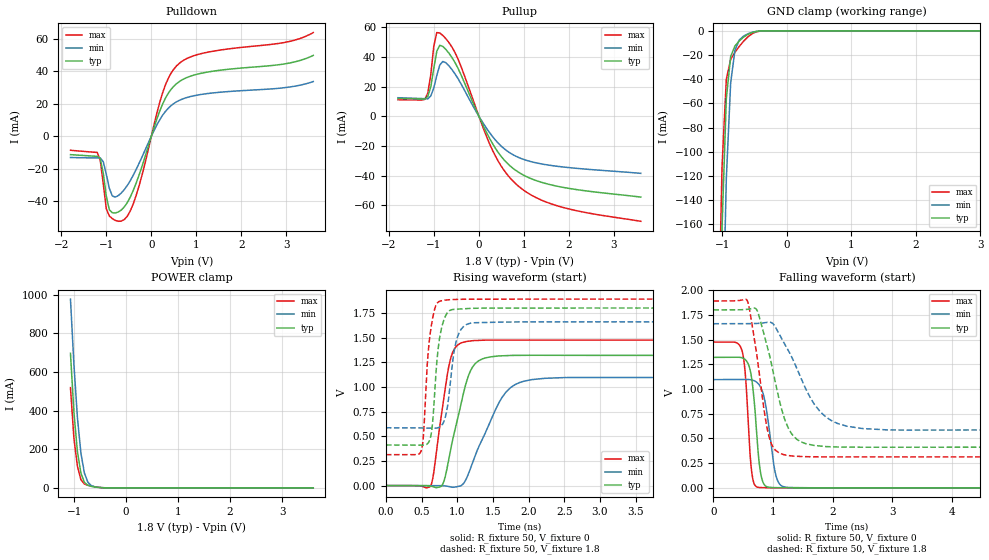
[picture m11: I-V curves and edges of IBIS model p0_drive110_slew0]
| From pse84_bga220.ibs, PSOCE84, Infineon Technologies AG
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[Model] p0_drive110_slew0
Model_type I/O
Polarity  Inverting
Enable   Active-High
Vinl  =  0.54
Vinh  =  1.26
Vmeas =  0.9
Cref  =  15pF
| Capacitance   typ   min   max
C_comp   1.253838e-12   1.215159e-12   1.300411e-12
| Variables   typ   min   max
[GND Clamp Reference]   0   0   0
[POWER Clamp Reference]   1.8   1.66   1.89
[Pulldown Reference]   0   0   0
[Pullup Reference]   1.8   1.66   1.89
[Temperature Range]   25   125   -40
[Voltage Range]   1.8   1.66   1.89
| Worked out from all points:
|   slope of the pulldown table from 0 to 0.27 V, typ, clamps not added: 12.9 ohm
|   slope of the pullup table from 0 to 0.27 V, typ, clamps not added: 16.3 ohm
|   GND clamp passes 1 mA (typ) near -0.51 V on its own axis
|   POWER clamp passes 1 mA (typ) near -0.47 V on its own axis
|   rising waveform, R_fixture 50, V_fixture 0: 20-80 % time 250ps typ, 406ps min, 174ps max; typ from 0 V to 1.32 V
|   rising waveform, R_fixture 50, V_fixture 1.8: 20-80 % time 98.2ps typ, 117ps min, 90.6ps max; typ from 0.411 V to 1.8 V
|   falling waveform, R_fixture 50, V_fixture 0: 20-80 % time 113ps typ, 152ps min, 89.3ps max; typ from 1.32 V to 0 V
|   falling waveform, R_fixture 50, V_fixture 1.8: 20-80 % time 335ps typ, 546ps min, 224ps max; typ from 1.8 V to 0.411 V
[GND Clamp]
| Voltage   I(typ)   I(min)   I(max)
-1.137V   -619.5mA   -754.2mA   -533mA
-1.07V    -361.2mA   -498.1mA   -281.3mA
-1.003V   -163.8mA   -277.7mA   -113mA
-936.6mV  -56.22mA   -122.3mA   -40.06mA
-869.7mV  -21.33mA   -43.3mA    -23.67mA
-802.8mV  -12.5mA    -15.96mA   -17.71mA
-735.9mV  -8.346mA   -7.675mA   -12.88mA
-669mV    -5.267mA   -4.349mA   -8.575mA
-535.2mV  -1.314mA   -1.207mA   -2.328mA
-401.4mV  -73.55uA   -132.2uA   -119.3uA
3.6V      0A         0A         0A
[POWER Clamp]
| Voltage   I(typ)   I(min)   I(max)
-1.07V    696.7mA    977.2mA    518.8mA
-1.003V   390.1mA    637.2mA    255.1mA
-936.6mV  187.1mA    363.9mA    112.4mA
-869.7mV  77.2mA     180.7mA    42.71mA
-802.8mV  28.89mA    77.43mA    19.98mA
-735.9mV  13.12mA    29.18mA    13.35mA
-669mV    7.754mA    11.55mA    8.954mA
-535.2mV  2.356mA    2.862mA    2.667mA
-334.5mV  34.33uA    127.4uA    15.58uA
3.6V      0A         0A         0A
[Pullup]
| Voltage   I(typ)   I(min)   I(max)
-1.8V     11.96mA    12.52mA    11.17mA
-1.204V   11.63mA    11.87mA    11.36mA
-1.07V    19.81mA    13.65mA    28.15mA
-1.003V   32.26mA    19.14mA    47.26mA
-936.6mV  43.85mA    27.48mA    56.38mA
-869.7mV  47.83mA    34.58mA    56.11mA
-735.9mV  45.06mA    36.08mA    52.29mA
-468.3mV  32.52mA    25.53mA    38.8mA
310.3mV   -18.74mA   -13.88mA   -23.33mA
806.9mV   -36.11mA   -26.63mA   -45.05mA
1.738V    -47.03mA   -33.62mA   -60.19mA
3.6V      -54.37mA   -38.39mA   -70.66mA
[Pulldown]
| Voltage   I(typ)   I(min)   I(max)
-1.8V     -11.4mA    -13.16mA   -8.708mA
-1.204V   -12.44mA   -13.38mA   -10.06mA
-1.137V   -13.75mA   -13.38mA   -14.91mA
-1.003V   -36.83mA   -23.35mA   -44.61mA
-936.6mV  -45.27mA   -32.05mA   -49.07mA
-869.7mV  -47.17mA   -36.79mA   -50.78mA
-669mV    -45.46mA   -34.98mA   -52.27mA
-401.4mV  -33.27mA   -23.95mA   -41.53mA
248.3mV   19.64mA    12.78mA    26.51mA
558.6mV   32.22mA    21.07mA    43.15mA
1.117V    38.69mA    25.66mA    50.78mA
3.6V      49.62mA    33.56mA    63.67mA
[Ramp]
dV/dt_r   0.791903/0.250198n  0.656961/0.40626n  0.884729/0.174201n
dV/dt_f   0.83321/0.335452n  0.644572/0.546477n  0.946064/0.22363n
R_load = 50
[Rising Waveform]
R_fixture = 50
V_fixture = 0
V_fixture_min = 0
V_fixture_max = 0
| Time   V(typ)   V(min)   V(max)
0s        11.48nV    820.1nV    4.127nV
625.1ps   -5.145mV   -5.381uV   -6.829mV
783.2ps   -1.996mV   -1.62mV    728.5mV
873.3ps   231.7mV    -7.82mV    1.174V
967.3ps   557.9mV    -15.47mV   1.394V
1.16ns    1.118V     123.1mV    1.464V
1.35ns    1.283V     464.5mV    1.474V
1.749ns   1.319V     993.7mV    1.475V
2.502ns   1.32V      1.095V     1.474V
50ns      1.32V      1.095V     1.475V
[Rising Waveform]
R_fixture = 50
V_fixture = 1.8
V_fixture_min = 1.66
V_fixture_max = 1.89
| Time   V(typ)   V(min)   V(max)
0s        411.3mV    585.7mV    313.2mV
492.7ps   409.1mV    583.6mV    346.3mV
527.9ps   409.4mV    582.7mV    514.2mV
602.5ps   441.1mV    581.6mV    1.42V
765.1ps   1.544V     598.9mV    1.871V
850.2ps   1.739V     744mV      1.881V
946.2ps   1.786V     1.309V     1.886V
1.125ns   1.795V     1.63V      1.889V
1.789ns   1.8V       1.658V     1.89V
50ns      1.8V       1.66V      1.89V
[Falling Waveform]
R_fixture = 50
V_fixture = 0
V_fixture_min = 0
V_fixture_max = 0
| Time   V(typ)   V(min)   V(max)
0s        1.32V      1.095V     1.475V
475.6ps   1.317V     1.096V     1.397V
537.6ps   1.295V     1.096V     1.135V
609ps     1.21V      1.095V     389.3mV
645.5ps   1.093V     1.091V     146.6mV
782.9ps   183.5mV    1.027V     3.184mV
873.4ps   19.23mV    848mV      1.671mV
1.053ns   2.057mV    115mV      719.4uV
1.296ns   753.8uV    3.568mV    293.1uV
50ns      11.46nV    883.3nV    4.128nV
[Falling Waveform]
R_fixture = 50
V_fixture = 1.8
V_fixture_min = 1.66
V_fixture_max = 1.89
| Time   V(typ)   V(min)   V(max)
0s        1.8V       1.66V      1.89V
558ps     1.805V     1.66V      1.902V
724.3ps   1.803V     1.663V     1.362V
870.4ps   1.505V     1.671V     704.3mV
956.7ps   1.3V       1.674V     468.8mV
1.162ns   755.8mV    1.49V      338.9mV
1.352ns   519.8mV    1.273V     320.6mV
1.878ns   417.8mV    720.3mV    313.2mV
2.914ns   410.9mV    586.2mV    313.3mV
50ns      411.3mV    585.7mV    313.2mV
